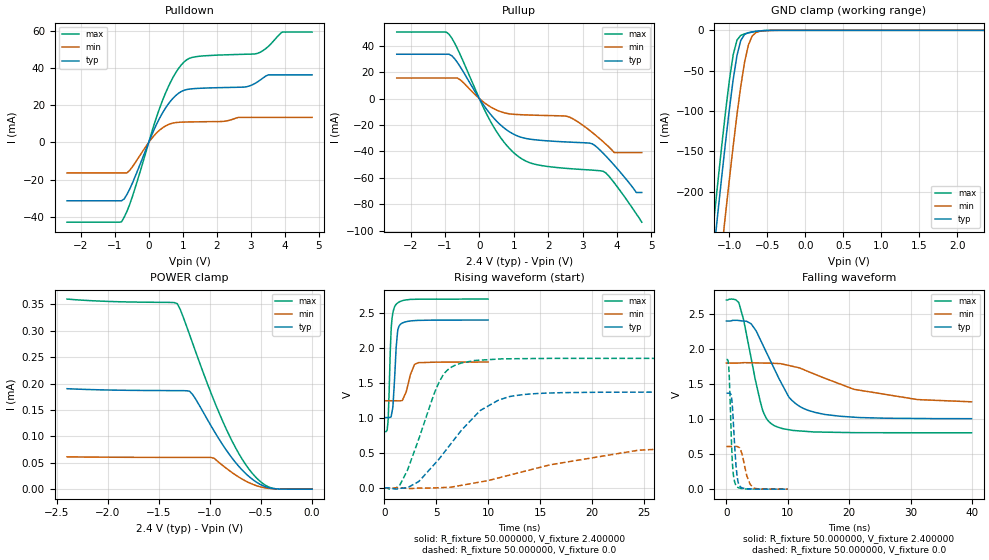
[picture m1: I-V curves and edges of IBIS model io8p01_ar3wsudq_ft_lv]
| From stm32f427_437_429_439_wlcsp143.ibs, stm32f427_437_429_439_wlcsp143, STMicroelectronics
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|   Model io8p01_ar3wsudq_ft_lv
[Model]  io8p01_ar3wsudq_ft_lv
Model_type I/O
Polarity   Non-Inverting
Enable   Active-Low
Vinl =   0.720000V
Vinh =   1.680000V
Vmeas =  1.200000V
Cref =   50.000000pF
Rref =   100.000000M
Vref =   0.0V
C_comp   3.720900pF   3.684200pF   3.822900pF
[Temperature Range]   25.000000   0.125000k   -40.000000
[Pullup Reference]   2.400000V   1.800000V   2.700000V
[Pulldown Reference]   0.0V   0.0V   0.0V
[POWER Clamp Reference]   2.400000V   1.800000V   2.700000V
[GND Clamp Reference]   0.0V   0.0V   0.0V
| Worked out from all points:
|   slope of the pulldown table from 0 to 0.36 V, typ, clamps not added: 25 ohm
|   slope of the pullup table from 0 to 0.36 V, typ, clamps not added: 27.7 ohm
|   GND clamp passes 1 mA (typ) near -0.62 V on its own axis
|   rising waveform, R_fixture 50.000000, V_fixture 2.400000: 20-80 % time 331ps typ, 645ps min, 264ps max; typ from 1.01 V to 2.4 V
|   rising waveform, R_fixture 50.000000, V_fixture 0.0: 20-80 % time 4.73ns typ, 11.9ns min, 2.67ns max; typ from 0 V to 1.37 V
|   falling waveform, R_fixture 50.000000, V_fixture 2.400000: 20-80 % time 4.88ns typ, 12.5ns min, 2.7ns max; typ from 2.4 V to 1.01 V
|   falling waveform, R_fixture 50.000000, V_fixture 0.0: 20-80 % time 594ps typ, 1.03ns min, 461ps max; typ from 1.37 V to 0 V
[Pulldown]
|Voltage   I(typ)   I(min)   I(max)
-2.4V     -31.47mA   -16.45mA   -43.01mA
-800mV    -31.47mA   -16.45mA   -42.85mA
-480mV    -21.98mA   -13.17mA   -29.21mA
80mV      3.63mA     1.966mA    5.014mA
480mV     18.16mA    8.738mA    26.02mA
800mV     25.38mA    10.72mA    37.77mA
1.12V     28.53mA    11.02mA    44.6mA
2.8V      29.84mA    13.51mA    47.53mA
3.2V      32.66mA    13.51mA    48.04mA
3.52V     36.44mA    13.51mA    51.84mA
3.92V     36.44mA    13.51mA    59.5mA
4.8V      36.44mA    13.51mA    59.5mA
[Pullup]
|Voltage   I(typ)   I(min)   I(max)
-2.4V     33.58mA    15.57mA    50.36mA
-960mV    33.58mA    15.57mA    50.36mA
-560mV    24.29mA    14.31mA    33.53mA
320mV     -11.75mA   -6.207mA   -17.08mA
960mV     -26.47mA   -11.82mA   -40.02mA
1.52V     -30.88mA   -12.51mA   -49.05mA
2.56V     -32.88mA   -13.52mA   -52.9mA
3.28V     -34.25mA   -25.64mA   -54.18mA
3.6V      -41.44mA   -32.74mA   -55.03mA
3.92V     -50.46mA   -40.9mA    -63.79mA
4.56V     -71.1mA    -40.9mA    -87.26mA
4.72V     -71.1mA    -40.9mA    -93.6mA
[GND_clamp]
|Voltage   I(typ)   I(min)   I(max)
-2.4V     -1.43A     -1.515A    -1.399A
-1.25V    -315.9mA   -407.2mA   -278.2mA
-1.2V     -270.1mA   -361.3mA   -232.1mA
-1.15V    -225mA     -316mA     -186.8mA
-1.1V     -180.9mA   -271.3mA   -142.7mA
-1.05V    -138.2mA   -227.5mA   -100.5mA
-950mV    -61.14mA   -143.6mA   -30.43mA
-900mV    -31.23mA   -104.7mA   -12.14mA
-850mV    -12.49mA   -69.4mA    -6.221mA
-750mV    -2.898mA   -18.35mA   -3.18mA
-600mV    -750.2uA   -1.218mA   -738.3uA
2.35V     0A         0A         0A
[POWER_clamp]
|Voltage   I(typ)   I(min)   I(max)
-2.4V     190.2uA    61.19uA    359.9uA
-1.32V    186.6uA    60.14uA    351.2uA
-1.29V    186.5uA    60.13uA    339.6uA
-1.2V     185.4uA    60.11uA    292.6uA
-1.17V    179.2uA    60.11uA    276.3uA
-960mV    110.2uA    58.62uA    167.5uA
-870mV    82.44uA    43.99uA    126.3uA
-750mV    50.58uA    26.92uA    78.64uA
-630mV    25.94uA    13.41uA    41.02uA
-510mV    9.22uA     4.527uA    14.97uA
-420mV    2.425uA    1.38uA     3.75uA
0V        0A         0A         0A
[Ramp]
| variable   typ   min   max
dV/dt_r  0.82224/4.72386n   0.36518/11.89627n   1.11114/2.66429n
dV/dt_f  0.83682/4.88809n   0.32346/13.40640n   1.13795/2.70298n
R_load = 50.000000
[Rising Waveform]
R_fixture= 50.000000
V_fixture= 2.400000
V_fixture_min= 1.800000
V_fixture_max= 2.700000
|time   V(typ)   V(min)   V(max)
0s        1.006V     1.247V     804.7mV
340.3ps   1.006V     1.247V     950.9mV
640.6ps   1.019V     1.247V     2.261V
820.8ps   1.188V     1.247V     2.51V
1.081ns   1.883V     1.247V     2.617V
1.281ns   2.26V      1.246V     2.646V
1.822ns   2.364V     1.285V     2.681V
2.883ns   2.392V     1.763V     2.696V
3.263ns   2.395V     1.791V     2.697V
9.97ns    2.4V       1.8V       2.7V
[Rising Waveform]
R_fixture= 50.000000
V_fixture= 0.0
V_fixture_min= 0.0
V_fixture_max= 0.0
|time   V(typ)   V(min)   V(max)
0s        177.7uV    72.88uV    448.7uV
1.522ns   -4.558mV   139.9uV    54.49mV
3.283ns   91.3mV     -1.149mV   693.1mV
5.205ns   405mV      3.698mV    1.495V
6.086ns   573.3mV    9.566mV    1.688V
7.367ns   818.4mV    37.04mV    1.785V
9.209ns   1.106V     85.61mV    1.826V
13.37ns   1.334V     234.4mV    1.848V
24.5ns    1.369V     540.7mV    1.852V
39.88ns   1.37V      609mV      1.852V
[Falling Waveform]
R_fixture= 50.000000
V_fixture= 2.400000
V_fixture_min= 1.800000
V_fixture_max= 2.700000
|time   V(typ)   V(min)   V(max)
0s        2.4V       1.8V       2.7V
2.002ns   2.407V     1.801V     2.665V
2.803ns   2.4V       1.805V     2.412V
4.004ns   2.362V     1.804V     1.876V
5.846ns   2.073V     1.8V       1.14V
7.768ns   1.721V     1.796V     908mV
10.57ns   1.275V     1.757V     842mV
14.41ns   1.095V     1.639V     816.4mV
20.82ns   1.027V     1.424V     806.5mV
39.88ns   1.006V     1.247V     804.7mV
[Falling Waveform]
R_fixture= 50.000000
V_fixture= 0.0
V_fixture_min= 0.0
V_fixture_max= 0.0
|time   V(typ)   V(min)   V(max)
0s        1.37V      609mV      1.852V
380.4ps   1.37V      609.1mV    1.736V
880.9ps   1.273V     608.9mV    543.4mV
1.121ns   955.3mV    608.6mV    210.2mV
1.481ns   429.3mV    609.3mV    65.8mV
1.762ns   165.9mV    609mV      32.06mV
2.122ns   51.18mV    592.9mV    16.15mV
3.323ns   5.987mV    186.4mV    3.21mV
4.505ns   2.283mV    13.72mV    1.528mV
9.97ns    177.7uV    72.88uV    448.7uV
